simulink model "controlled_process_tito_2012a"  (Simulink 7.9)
settings: Solver=ode3  StartTime=0.0  StopTime=simopt.Tf  FixedStep=simopt.h  RelTol=1e-3
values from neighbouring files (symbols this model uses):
  simopt = []    [setParams.m]
libraries: cstblocks x4

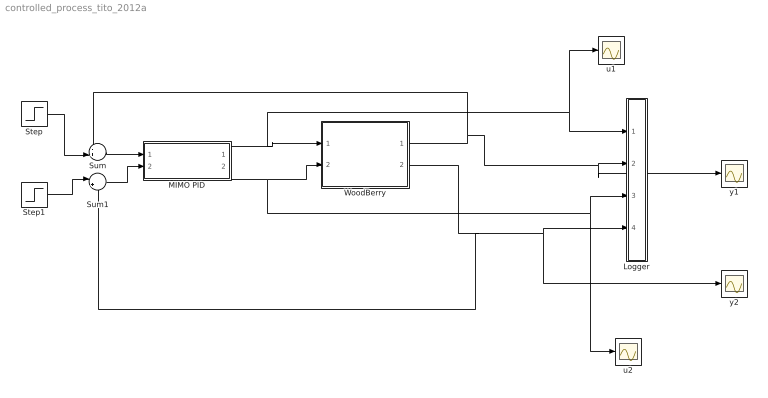
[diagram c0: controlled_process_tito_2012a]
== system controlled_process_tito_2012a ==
  Logger : Subsystem
  MIMO PID : Subsystem
  Step : Step  Time=0  Before=2  After=2  SampleTime=simopt.h
  Step1 : Step  Time=100  Before=3  SampleTime=simopt.h
  Sum : Sum  Inputs=-+|
  Sum1 : Sum  Inputs=|+-
  WoodBerry : Subsystem
  u1 : Scope
  u2 : Scope
  y1 : Scope
  y2 : Scope
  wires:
  MIMO PID/1(u1) -> Logger/1(u1), u1/1, WoodBerry/1(u1)
  MIMO PID/2(u2) -> Logger/3(u2), u2/1, WoodBerry/2(u2)
  WoodBerry/1(y1) -> Logger/2(y1), y1/1, Sum/1
  WoodBerry/2(y2) -> Logger/4(y2), y2/1, Sum1/2
  Step/1 -> Sum/2
  Step1/1 -> Sum1/1
  Sum/1 -> MIMO PID/1(e1)
  Sum1/1 -> MIMO PID/2(e2)

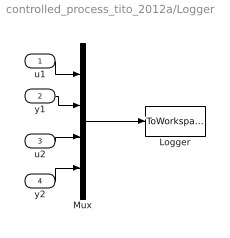
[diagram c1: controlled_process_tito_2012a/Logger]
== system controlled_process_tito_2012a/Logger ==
  u1 : Inport  SampleTime=simopt.h
  y1 : Inport  Port=2  SampleTime=simopt.h
  u2 : Inport  Port=3  SampleTime=simopt.h
  y2 : Inport  Port=4  SampleTime=simopt.h
  Logger : ToWorkspace  VariableName=simout  SampleTime=simopt.h  SaveFormat=Structure With Time
  Mux : Mux
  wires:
  Mux/1 -> Logger/1
  u1/1 -> Mux/1
  y1/1 -> Mux/2
  u2/1 -> Mux/3
  y2/1 -> Mux/4

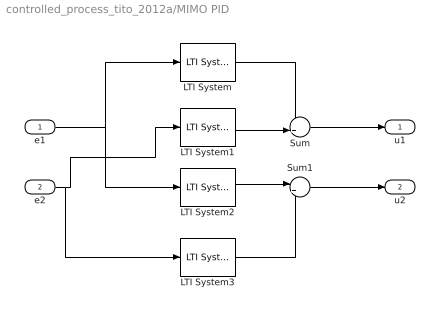
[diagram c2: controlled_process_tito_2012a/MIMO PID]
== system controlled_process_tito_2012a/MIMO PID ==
  e1 : Inport
  e2 : Inport  Port=2
  LTI System : cstblocks/LTI System  sys=C11  IC=[]
  LTI System1 : cstblocks/LTI System  sys=C12  IC=[]
  LTI System2 : cstblocks/LTI System  sys=C21  IC=[]
  LTI System3 : cstblocks/LTI System  sys=C22  IC=[]
  Sum : Sum  Inputs=++|
  Sum1 : Sum  Inputs=|++
  u1 : Outport
  u2 : Outport  Port=2
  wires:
  e1/1 -> LTI System/1, LTI System2/1
  e2/1 -> LTI System1/1, LTI System3/1
  LTI System3/1 -> Sum1/2
  Sum1/1 -> u2/1
  LTI System/1 -> Sum/1
  Sum/1 -> u1/1
  LTI System2/1 -> Sum1/1
  LTI System1/1 -> Sum/2

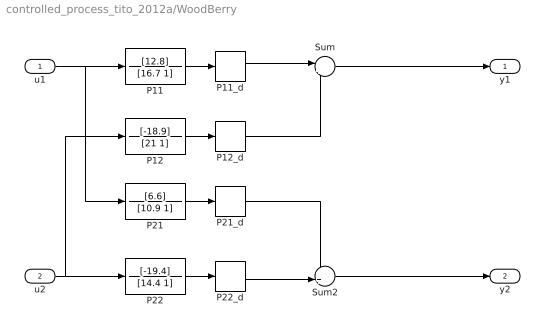
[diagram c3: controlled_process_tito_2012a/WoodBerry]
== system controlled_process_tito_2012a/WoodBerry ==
  u1 : Inport
  u2 : Inport  Port=2
  P11 : TransferFcn  Numerator=[12.8]  Denominator=[16.7 1]
  P11_d : TransportDelay
  P12 : TransferFcn  Numerator=[-18.9]  Denominator=[21 1]
  P12_d : TransportDelay  DelayTime=3
  P21 : TransferFcn  Numerator=[6.6]  Denominator=[10.9 1]
  P21_d : TransportDelay  DelayTime=7
  P22 : TransferFcn  Numerator=[-19.4]  Denominator=[14.4 1]
  P22_d : TransportDelay  DelayTime=3
  Sum : Sum  Inputs=|++
  Sum2 : Sum  Inputs=++|
  y1 : Outport
  y2 : Outport  Port=2
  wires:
  Sum2/1 -> y2/1
  P22_d/1 -> Sum2/2
  P22/1 -> P22_d/1
  P21_d/1 -> Sum2/1
  P21/1 -> P21_d/1
  u2/1 -> P22/1, P12/1
  P12_d/1 -> Sum/2
  P12/1 -> P12_d/1
  u1/1 -> P21/1, P11/1
  Sum/1 -> y1/1
  P11_d/1 -> Sum/1
  P11/1 -> P11_d/1
